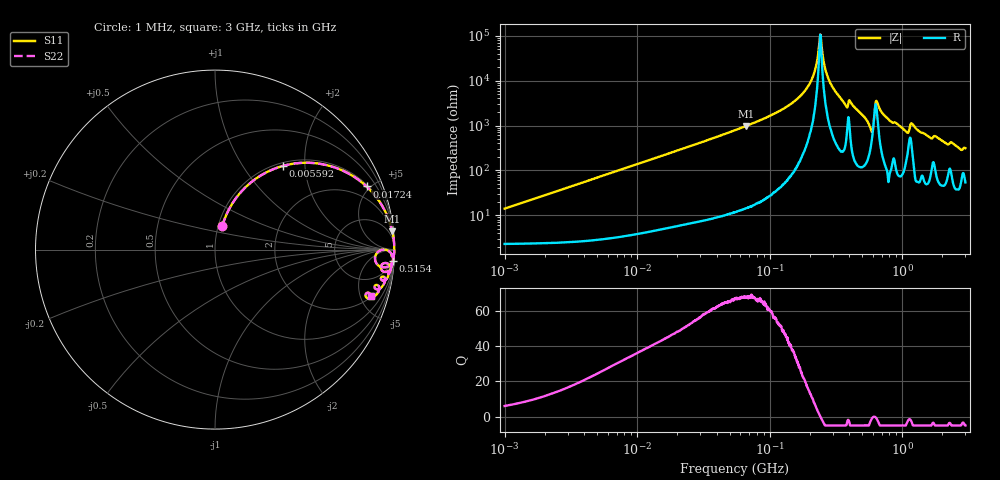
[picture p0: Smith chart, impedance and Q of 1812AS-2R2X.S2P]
!s-Parameter Generated by FASTRON Sdn. Bhd.
!FASTRON P/N : 1812AS-2R2X
!Keysight Technologies,E4991B,MY54100416,A.01.15
!Date created: Fri Oct 13 15:39:41 2023
!Version  : Rev00 Fri Oct 13 15:39:41 2023
!Data & Calibration Information:
!Freq	S11	S21	S12	S22
!PortZ  Port1:50+j0  Port2:50+j0
!When reading, reference impedance value at option line is always used.
! Remarks : This data is being provided solely for informational purposes.
# Hz S dB R 50
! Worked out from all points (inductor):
!   1601 points, 1 MHz to 3 GHz, reference 50 ohm
!   read as one part in series: L = 2.22 uH near 1.041 MHz
!   highest Q = 68 at 66.58 MHz (marker M1), where L = 2.33 uH
!   self-resonance near 240.9 MHz
!   S11 on the Smith chart (normalised r, x): 1 MHz: 1.05, +0.28; 5.592 MHz: 1.06, +1.55; 17.24 MHz: 1.11, +4.75; 515.4 MHz: 3, -31; 3 GHz: 2.08, -6.15
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1000000  -17.28 72.8  -0.28 -7.8  -0.28 -7.8  -17.28 72.8
3804036  -6.78 59.9  -1.25 -27.2  -1.25 -27.2  -6.78 59.9
5592179  -4.41 50.9  -2.20 -37.0  -2.20 -37.0  -4.41 50.9
1.447069e7  -1.05 26.3  -7.06 -62.3  -7.06 -62.3  -1.05 26.3
1.724056e7  -0.78 22.6  -8.30 -66.1  -8.30 -66.1  -0.78 22.6
5.477226e7  -0.09 7.3  -17.97 -81.9  -17.97 -81.9  -0.09 7.3
6.657566e7  -0.06 5.8  -19.85 -83.3  -19.85 -83.3  -0.06 5.8
1.453231e8  -0.01 1.9  -29.72 -86.7  -29.72 -86.7  -0.01 1.9
2.083556e8  -0.01 0.5  -40.67 -84.3  -40.67 -84.3  -0.01 0.5
2.421036e8  -0.01 -0.0  -60.26 12.7  -60.26 12.7  -0.01 -0.0
2.675872e8  -0.01 -0.4  -43.49 80.6  -43.49 80.6  -0.01 -0.4
3.017325e8  -0.01 -0.8  -36.62 84.5  -36.62 84.5  -0.01 -0.8
3.72303e8  -0.04 -1.9  -29.33 81.1  -29.33 81.1  -0.04 -1.9
4.094372e8  -0.04 -1.7  -30.30 80.6  -30.30 80.6  -0.04 -1.7
5.154121e8  -0.06 -3.6  -24.02 81.9  -24.02 81.9  -0.06 -3.6
5.870266e8  -0.69 -5.9  -18.11 49.4  -18.11 49.4  -0.69 -5.9
6.488164e8  -0.13 -1.5  -30.38 59.0  -30.38 59.0  -0.13 -1.5
7.925923e8  -0.05 -4.2  -22.60 83.1  -22.60 83.1  -0.05 -4.2
1.070143e9  -0.32 -7.4  -17.62 70.5  -17.62 70.5  -0.32 -7.4
1.194682e9  -0.21 -5.1  -20.86 71.9  -20.86 71.9  -0.21 -5.1
1.613037e9  -0.32 -10.2  -15.01 73.2  -15.01 73.2  -0.32 -10.2
3e9  -0.84 -16.6  -10.73 63.4  -10.73 63.4  -0.84 -16.6
